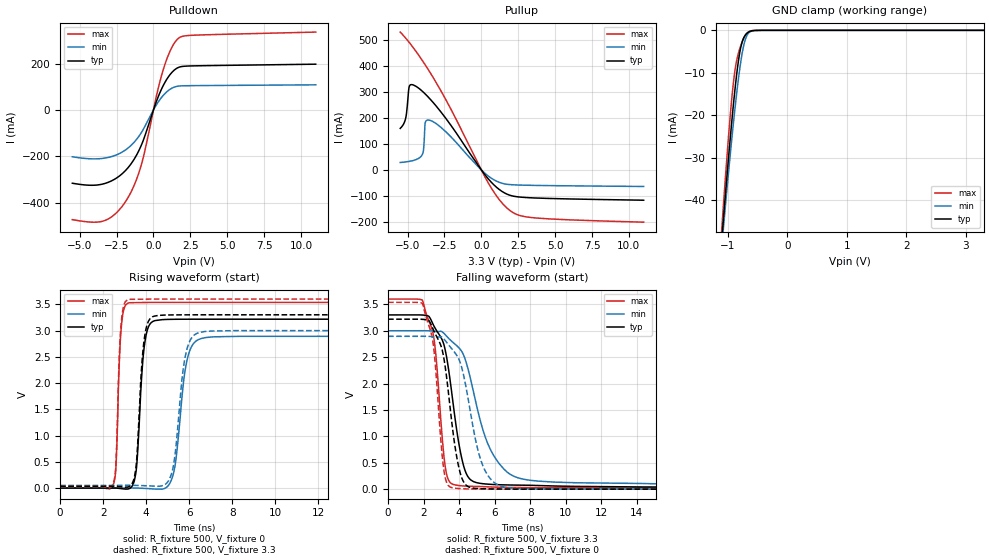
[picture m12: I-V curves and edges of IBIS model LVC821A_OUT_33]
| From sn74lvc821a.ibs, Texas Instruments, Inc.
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[Model]   LVC821A_OUT_33
Model_type  3-state
Enable   Active-Low
Vref =   0
Rref =   500
Cref =   50p
Vmeas =   1.5
| variable   typ   min   max
C_comp   6.47pF   5.76pF   7.74pF
| C_pullup   8.61pF   7.74pF   9.74pF
| C_pulldown   12.41pF   7.74pF   18.95pF
| C_tri-state   6.47pF   5.76pF   7.74pF
[Temperature Range]   40   100   -40
| Ambient temperature   25   85   -40
[Voltage range]   3.3   3   3.6
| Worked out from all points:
|   slope of the pulldown table from 0 to 0.495 V, typ, clamps not added: 5.98 ohm
|   slope of the pullup table from 0 to 0.495 V, typ, clamps not added: 13.7 ohm
|   GND clamp passes 1 mA (typ) near -0.70 V on its own axis
|   rising waveform, R_fixture 500, V_fixture 0: 20-80 % time 281ps typ, 448ps min, 175ps max; typ from 0 V to 3.22 V
|   falling waveform, R_fixture 500, V_fixture 3.3: 20-80 % time 874ps typ, 1.54ns min, 544ps max; typ from 3.3 V to 0.035 V
|   rising waveform, R_fixture 500, V_fixture 3.3: 20-80 % time 276ps typ, 433ps min, 173ps max; typ from 0.034 V to 3.3 V
|   falling waveform, R_fixture 500, V_fixture 0: 20-80 % time 761ps typ, 1.06ns min, 521ps max; typ from 3.22 V to 0 V
[GND Clamp]
| LVC821A_OUT_33
|   Voltage   I(typ)   I(min)   I(max)
-5.5V     -1.089A    -967.7mA   -1.248A
-1.1V     -48.78mA   -50.46mA   -46.17mA
-1.07V    -43.53mA   -45.73mA   -40.17mA
-1V       -31.73mA   -35.04mA   -26.91mA
-955mV    -24.58mA   -28.48mA   -19.22mA
-910mV    -17.9mA    -22.22mA   -12.67mA
-875mV    -13.15mA   -17.64mA   -8.877mA
-820mV    -6.936mA   -11.12mA   -5.241mA
-770mV    -3.231mA   -6.228mA   -3.071mA
-710mV    -1.17mA    -2.286mA   -1.248mA
-635mV    -274.4uA   -424.5uA   -227uA
3.3V      71.7pA     13.58nA    66.83pA
[Pulldown]
| LVC821A_OUT_33
|   Voltage   I(typ)   I(min)   I(max)
-5.5V     -316.2mA   -202.2mA   -473.2mA
-3.265V   -316.6mA   -207.4mA   -476.1mA
-2.465V   -292.1mA   -192.8mA   -440.8mA
-1.73V    -249.6mA   -164.6mA   -378.7mA
-1.22V    -203mA     -132.7mA   -311.4mA
-785mV    -146.5mA   -94.08mA   -228.2mA
245mV     44.12mA    26.7mA     72.48mA
715mV     111.4mA    66.3mA     184mA
1.215V    159.3mA    92.45mA    265.8mA
1.705V    183.5mA    102.8mA    309.6mA
2.755V    190mA      104.8mA    322.3mA
11V       197.3mA    108.2mA    335.7mA
[Pullup]
| LVC821A_OUT_33
|   Voltage   I(typ)   I(min)   I(max)
-5.5V     160.4mA    28.92mA    531.9mA
-5.125V   201.1mA    31.13mA    508.1mA
-4.88V    323.4mA    33.24mA    491mA
-4.435V   322.7mA    39.82mA    457.5mA
-3.975V   302.2mA    63.53mA    419.9mA
-3.905V   298.4mA    87.69mA    413.9mA
-3.805V   292.9mA    182.2mA    405.2mA
-3.495V   274.6mA    191.7mA    377.5mA
490mV     -35.88mA   -24.34mA   -52.28mA
1.9V      -96.96mA   -56.25mA   -155mA
3.67V     -108.2mA   -59.57mA   -185.1mA
11V       -116.7mA   -63.69mA   -201.5mA
[Ramp]
| LVC821A_OUT_33
| variable   typ   min   max
dV/dt_r   1.94/2.98E-10   1.75/4.57E-10   2.13/1.85E-10
dV/dt_f   1.96/8.79E-10   1.77/1.55E-09   2.15/5.47E-10
R_load = 500
[Rising Waveform]
| LVC821A_OUT_33
R_fixture =   500
C_fixture =   0
L_fixture =   0
V_fixture =   0
V_fixture_min = 0
V_fixture_max = 0
|   Time   V(typ)   V(min)   V(max)
0s        472.5pV    747.4pV    297.5pV
2.475ns   1.554mV    135.9uV    67.98mV
2.83ns    -9.871mV   1.35mV     2.99V
3.155ns   -18.33mV   1.658mV    3.524V
3.965ns   2.836V     -6.977mV   3.535V
4.405ns   3.189V     -18.77mV   3.536V
5.24ns    3.214V     228.2mV    3.537V
5.89ns    3.216V     2.41V      3.537V
6.585ns   3.216V     2.851V     3.537V
29.99ns   3.217V     2.891V     3.537V
[Falling Waveform]
| LVC821A_OUT_33
R_fixture =   500
C_fixture =   0
L_fixture =   0
V_fixture =   3.3
V_fixture_min = 3
V_fixture_max = 3.6
|   Time   V(typ)   V(min)   V(max)
0s        3.3V       3V         3.6V
1.96ns    3.297V     3.001V     3.554V
2.6ns     3.078V     2.989V     2.81V
3.115ns   2.765V     2.961V     724.4mV
3.675ns   1.585V     2.773V     89.18mV
4.125ns   618.5mV    2.619V     63.88mV
4.56ns    206.8mV    2.198V     55.38mV
5.715ns   92.63mV    783.2mV    42.51mV
7.315ns   76.66mV    214.4mV    31.62mV
29.99ns   34.63mV    58.11mV    22.79mV
[Rising Waveform]
| LVC821A_OUT_33
R_fixture =   500
C_fixture =   0
L_fixture =   0
V_fixture =   3.3
V_fixture_min = 3
V_fixture_max = 3.6
|   Time   V(typ)   V(min)   V(max)
0s        34.13mV    50.9mV     22.72mV
2.465ns   35.6mV     51.03mV    86.3mV
2.825ns   24.99mV    52.18mV    3.059V
3.15ns    19.89mV    52.36mV    3.589V
3.925ns   2.869V     45.14mV    3.598V
4.38ns    3.275V     36.75mV    3.599V
5.19ns    3.298V     286.3mV    3.6V
5.815ns   3.3V       2.495V     3.6V
6.48ns    3.3V       2.964V     3.6V
29.99ns   3.3V       3V         3.6V
[Falling Waveform]
| LVC821A_OUT_33
R_fixture =   500
C_fixture =   0
L_fixture =   0
V_fixture =   0
V_fixture_min = 0
V_fixture_max = 0
|   Time   V(typ)   V(min)   V(max)
0s        3.219V     2.895V     3.538V
1.96ns    3.216V     2.895V     3.492V
2.545ns   3.022V     2.887V     2.738V
3.015ns   2.673V     2.881V     747.5mV
3.525ns   1.444V     2.683V     36.32mV
3.905ns   537.1mV    2.512V     13.57mV
4.295ns   114.3mV    2.089V     6.626mV
5.255ns   8.68mV     516.1mV    2.56mV
6.41ns    2.657mV    51.07mV    1.441mV
29.99ns   80.54uV    497.3uV    51.03uV
